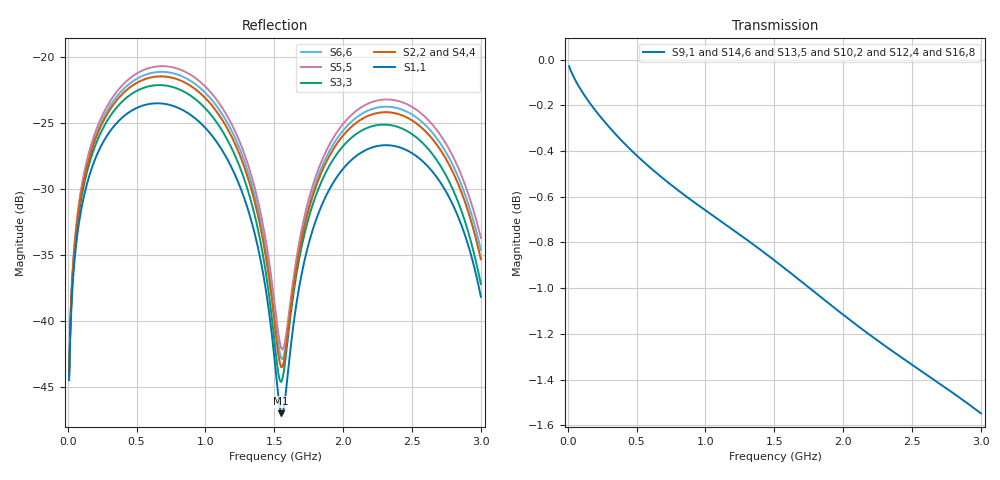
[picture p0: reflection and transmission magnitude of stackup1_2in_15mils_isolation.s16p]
! Touchstone file from project
# GHZ S RI R 50.000000
! Modal data exported
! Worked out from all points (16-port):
!   300 points, 10 MHz to 3 GHz, reference 50 ohm
!   strongest paths, dB at 10 MHz, 760 MHz, 1.51 GHz, 2.26 GHz, 3 GHz:
!     S9,1: 0.0, -0.6, -0.9, -1.2, -1.5
!     S14,6: 0.0, -0.6, -0.9, -1.3, -1.6
!     S13,5: 0.0, -0.6, -0.9, -1.3, -1.6
!     S10,2: 0.0, -0.6, -0.9, -1.3, -1.6
!     S12,4: 0.0, -0.6, -0.9, -1.3, -1.6
!     S16,8: 0.0, -0.6, -0.9, -1.2, -1.6
!   lowest |S11| = -47.0 dB at 1.55 GHz (marker M1), VSWR 1.01, Z = 50.4 - j0.189 ohm
!   |S11| at or under -10 dB: start of sweep to end of sweep
